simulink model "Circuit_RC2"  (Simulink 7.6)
settings: Solver=ode15s  StartTime=0.0  StopTime=10.0  RelTol=1e-3
InitFcn:
  | R=1e3;
  | C=1e-3;
  | U0=5;
StopFcn:
  | load circuit_RC.mat
  | plot(y(1,:),y(2,:))
  | title('Tension aux bornes de C, courant dans le circuit RC')
  | grid
  | %axis([0 10 -0.5 5.5])
libraries: fl_lib x5, nesl_utility x3

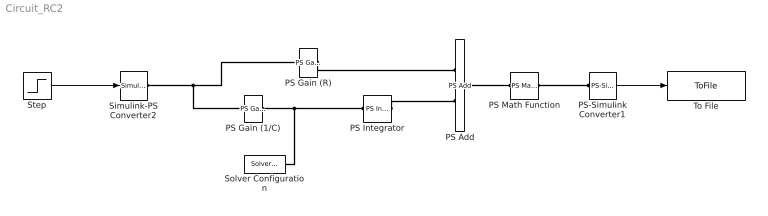
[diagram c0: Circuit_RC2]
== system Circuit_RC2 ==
  PS Add : fl_lib/Physical Signals/Functions/PS Add  DialogController=NetworkEngine.DynNeDlgSource  SystemSampleTime=-1  LocalVarLogging=[]
  PS Gain (1/C) : fl_lib/Physical Signals/Functions/PS Gain  DialogController=NetworkEngine.DynNeDlgSource  SystemSampleTime=-1  gain=1/C  LocalVarLogging=[]
  PS Gain (R) : fl_lib/Physical Signals/Functions/PS Gain  DialogController=NetworkEngine.DynNeDlgSource  SystemSampleTime=-1  gain=R  LocalVarLogging=[]
  PS Integrator : fl_lib/Physical Signals/Linear Operators/PS Integrator  DialogController=NetworkEngine.DynNeDlgSource  SystemSampleTime=-1  x0=0  x_Log=off  LocalVarNames=|x  LocalVarDescs=|x  LocalVarLogging=0
  PS Math Function : fl_lib/Physical Signals/Functions/PS Math Function  DialogController=NetworkEngine.DynNeDlgSource  SystemSampleTime=-1  fcn_choice=9  LocalVarLogging=[]
  PS-Simulink Converter1 : nesl_utility/PS-Simulink Converter  DialogController=NetworkEngine.DynNeUtilDlgSource  SystemSampleTime=-1  PhysicalDomain=network_engine_domain  LeftPortType=input  RightPortType=output  SubClassName=ps_output  Unit=1  AffineConversion=off
  Simulink-PS Converter2 : nesl_utility/Simulink-PS Converter  DialogController=NetworkEngine.DynNeUtilDlgSource  SystemSampleTime=-1  PhysicalDomain=network_engine_domain  LeftPortType=input  RightPortType=output  SubClassName=ps_input  Unit=1  AffineConversion=off  InputFilterTimeConstant=.001  UdotUserProvided=0
  Solver Configuration : nesl_utility/Solver Configuration  DialogController=NetworkEngine.DynNeUtilDlgSource  SystemSampleTime=-1  PhysicalDomain=network_engine_domain  LeftPortType=input  RightPortType=generic  SubClassName=solver  Accelerate=off  Profile=off  ResidualTolerance=1e-9  MaxNonlinIter=12  MaxModeIter=2  DoFixedCost=off  UseLocalSampling=off  DoDC=off  LinearAlgebra=Sparse  LocalSolverSampleTime=.001  LocalSolverChoice=NE_BACKWARD_EULER_ADVANCER  UseLocalSolver=off
  Step : Step  Time=0  After=U0  SampleTime=0
  To File : ToFile  Filename=circuit_RC.mat  MatrixName=y
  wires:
  Step/1 -> Simulink-PS Converter2/1
  PS-Simulink Converter1/1 -> To File/1
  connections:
  Simulink-PS Converter2/RConn1 -- PS Gain (R)/LConn1 -- PS Gain (1/C)/LConn1
  PS Integrator/RConn1 -- PS Add/LConn2
  PS Gain (1/C)/RConn1 -- PS Integrator/LConn1 -- Solver Configuration/RConn1
  PS Gain (R)/RConn1 -- PS Add/LConn1
  PS Math Function/RConn1 -- PS-Simulink Converter1/LConn1
  PS Add/RConn1 -- PS Math Function/LConn1
